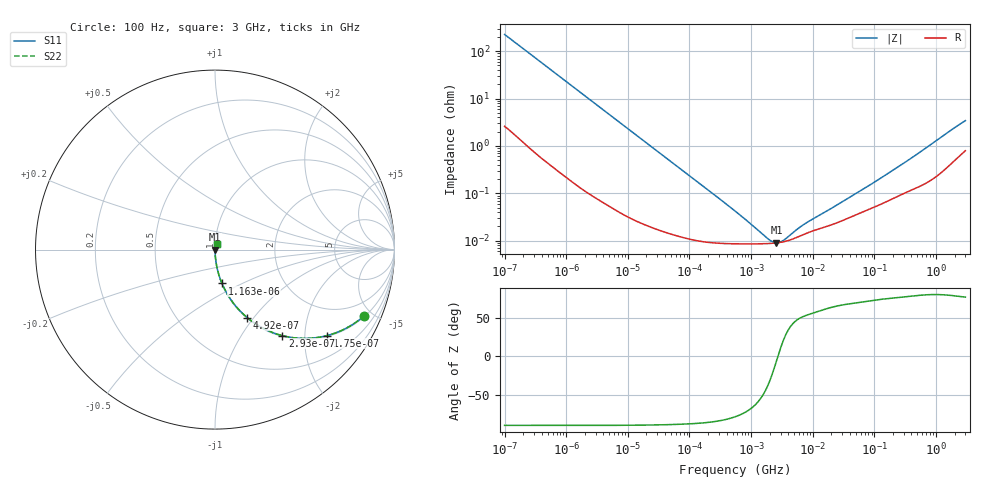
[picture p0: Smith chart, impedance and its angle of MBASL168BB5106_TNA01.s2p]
! MBASL168BB5106_TNA01  S-PARAMETER MODEL  ( Standard Model )
! Model Generated by TAIYO YUDEN Corporation (http://www.ty-top.com)
! Version 2.0
! TAIYO YUDEN Control No. 240306
! Copyright(c) 2012 TAIYO YUDEN CO.,LTD. All Rights Reserved.
! Product Description (link to TY-COMPAS)
! https://ds.yuden.co.jp/TYCOMPAS/or/detail?pn=MBASL168BB5106MTNA01&u=M
! Products Name : Multilayer Ceramic Capacitors
! Characteristics :
!  Capacitance : 10 [uF] , Rated Voltage : 10 [V] , TCC : X5R
!  Case Size : 1.6 x 0.8 / 0.063 x 0.031 [mm/inch] , Thickness : 0.8 / 0.031 [mm/inch]
!  (Conditions: Temperature = 25 [degC] , DC Bias Voltage = 0 [V])
! External Node Assignments :
!  1  o---| |---o  2
! GND o---------o GND
! Frequency Range : 100Hz  -  3GHz  [ 401 STEP ]
# MHZ S RI R 50
! Freq[MHz].  S11 Real  S11 Imag  S21 Real  S21 Imag  S12 Real  S12 Imag  S22 Real  S22 Imag
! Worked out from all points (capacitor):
!   401 points, 100 Hz to 3 GHz, reference 50 ohm
!   read as one part in series: C = 7.05 uF near 109 Hz
!   lowest |Z| = 9.05 mohm at 2.579 MHz (marker M1)
!   series resonance near 2.721 MHz, so ESL is about 490 pH
!   S11 on the Smith chart (normalised r, x): 100 Hz: 1.05, -4.50; 175 Hz: 1.03, -2.59; 293 Hz: 1.02, -1.55; 492 Hz: 1.01, -0.93; 1.163 kHz: 1.00, -0.39; 3 GHz: 1.02, +0.07
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0.0001  0.8324 -0.3678  0.1676 0.3678  0.1676 0.3678  0.8324 -0.3678
0.000124  0.7654 -0.4181  0.2346 0.4181  0.2346 0.4181  0.7654 -0.4181
0.000175  0.6244 -0.4789  0.3756 0.4789  0.3756 0.4789  0.6244 -0.4789
0.000227  0.5002 -0.4949  0.4998 0.4949  0.4998 0.4949  0.5002 -0.4949
0.000293  0.3757 -0.4794  0.6243 0.4794  0.6243 0.4794  0.3757 -0.4794
0.000492  0.1789 -0.3785  0.8211 0.3785  0.8211 0.3785  0.1789 -0.3785
0.000724  0.0925 -0.285  0.9075 0.285  0.9075 0.285  0.0925 -0.285
0.001163  0.0389 -0.1887  0.9611 0.1887  0.9611 0.1887  0.0389 -0.1887
0.001788  0.0173 -0.1258  0.9827 0.1258  0.9827 0.1258  0.0173 -0.1258
0.005476  0.00226 -0.042  0.9977 0.042  0.9977 0.042  0.00226 -0.042
0.031977  0.00022 -0.0073  0.9998 0.0073  0.9998 0.0073  0.00022 -0.0073
0.547723  8.62e-05 -0.000416  0.9999 0.000416  0.9999 0.000416  8.62e-05 -0.000416
1.908323  8.72e-05 -6.36e-05  0.9999 6.36e-05  0.9999 6.36e-05  8.72e-05 -6.36e-05
2.171352  8.81e-05 -4e-05  0.9999 4e-05  0.9999 4e-05  8.81e-05 -4e-05
2.579298  9e-05 -9.38e-06  0.9999 9.38e-06  0.9999 9.38e-06  9e-05 -9.38e-06
3.486191  9.62e-05 4.36e-05  0.9999 -4.36e-05  0.9999 -4.36e-05  9.62e-05 4.36e-05
6.10039  0.000124 0.000144  0.9999 -0.000144  0.9999 -0.000144  0.000124 0.000144
9.794414  0.000159 0.000233  0.9998 -0.000233  0.9998 -0.000233  0.000159 0.000233
59.714  0.000388 0.00107  0.9996 -0.00107  0.9996 -0.00107  0.000388 0.00107
175.1444  0.00072 0.00265  0.9993 -0.00265  0.9993 -0.00265  0.00072 0.00265
1950.712  0.00527 0.023  0.9947 -0.023  0.9947 -0.023  0.00527 0.023
3000  0.00893 0.0327  0.9911 -0.0327  0.9911 -0.0327  0.00893 0.0327
